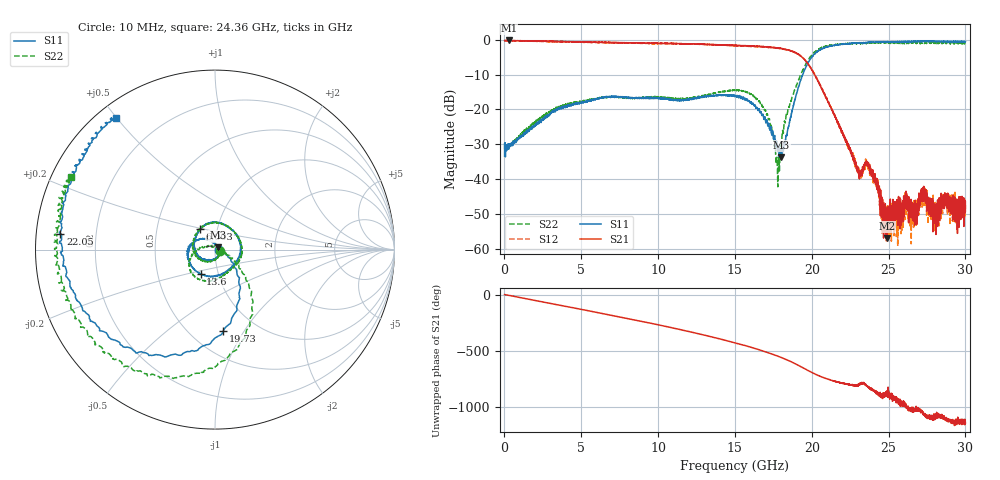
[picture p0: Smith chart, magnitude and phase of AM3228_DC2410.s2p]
!Agilent Technologies,E8364B,MY43040894,A.07.50.67
!Agilent E8364B: A.07.50.67
!Date: Thursday, April 11, 2024 13:26:10
!Correction: S11(Full 2 Port(1,2))
!S21(Full 2 Port(1,2))
!S12(Full 2 Port(1,2))
!S22(Full 2 Port(1,2))
!S2P File: Measurements: S11, S21, S12, S22:
# Hz S  dB  R 50
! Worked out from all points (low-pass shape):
!   6401 points, 10 MHz to 30 GHz, reference 50 ohm
!   highest |S21| = -0.20 dB at 295.8 MHz (marker M1); lowest = -57.1 dB at 24.88 GHz (marker M2)
!   |S21| within 3 dB of the highest: start of sweep to 18.67 GHz
!   lowest |S11| = -33.8 dB at 18.02 GHz (marker M3), VSWR 1.04, Z = 51.6 + j1.33 ohm
!   |S11| at or under -10 dB: start of sweep to 19.42 GHz
!   |S22| runs from -42.2 to -0.7 dB; largest |S21 - S12| = 0.035
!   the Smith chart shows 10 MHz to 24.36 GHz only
!   S11 on the Smith chart (normalised r, x): 10 MHz: 1.04, -0.01; 6.003 GHz: 0.83, +0.20; 13.6 GHz: 0.82, -0.23; 19.73 GHz: 0.71, -0.81; 22.05 GHz: 0.07, +0.05; 24.36 GHz: 0.05, +0.50
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1e7  -33.44 -9.6  -0.25 0.3  -0.42 -0.8  -31.44 -11.7
2.958422e8  -30.21 -19.4  -0.20 -7.7  -0.32 -8.2  -30.29 -20.2
2.751273e9  -21.91 -133.9  -0.39 -72.1  -0.52 -72.5  -21.10 -130.9
5.009895e9  -18.10 154.5  -0.64 -131.7  -0.74 -131.7  -17.65 157.6
6.003314e9  -16.95 125.3  -0.72 -157.9  -0.81 -158.0  -17.00 124.8
7.849573e9  -16.60 70.9  -0.86 152.7  -0.97 152.5  -16.68 61.2
1.000979e10  -16.70 3.4  -1.05 92.0  -1.09 92.0  -16.50 -11.2
1.20388e10  -17.11 -68.3  -1.18 31.1  -1.25 31.1  -16.83 -61.4
1.359922e10  -15.97 -120.1  -1.35 -19.2  -1.48 -19.0  -15.44 -89.8
1.5005e10  -16.31 -167.0  -1.65 -68.0  -1.73 -68.2  -14.47 -122.9
1.637329e10  -19.48 149.0  -1.81 -120.9  -1.98 -120.5  -16.82 -159.4
1.724488e10  -25.46 121.0  -2.08 -159.2  -2.24 -158.6  -22.71 168.9
1.777439e10  -31.77 81.3  -2.32 174.6  -2.45 175.5  -38.60 102.0
1.802274e10  -33.80 39.1  -2.53 161.7  -2.60 162.3  -30.80 -1.9
1.892244e10  -17.07 -41.2  -3.67 107.2  -3.69 107.9  -14.18 -38.8
1.972842e10  -6.81 -84.3  -6.78 48.9  -6.74 49.3  -6.08 -69.8
2.00049e10  -4.90 -100.1  -8.65 28.8  -8.60 28.5  -4.34 -83.4
2.205265e10  -1.26 174.2  -27.20 -67.1  -26.92 -70.1  -1.13 -161.4
2.436282e10  -0.71 126.8  -44.97 -158.5  -45.36 -173.2  -0.92 152.6
2.488296e10  -0.73 117.5  -57.05 -176.8  -49.88 -153.0  -0.90 143.2
2.500479e10  -0.70 115.4  -53.19 -173.1  -52.51 -157.7  -0.97 140.9
3e10  -0.51 43.2  -46.56 -60.7  -47.58 -48.2  -0.88 72.7
